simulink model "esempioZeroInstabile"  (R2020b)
settings: Solver=FixedStepAuto  StartTime=0.0  StopTime=30  FixedStep=0.01  RelTol=1e-3

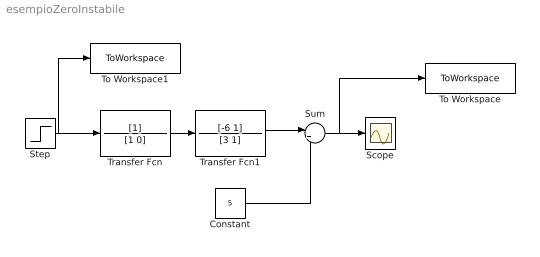
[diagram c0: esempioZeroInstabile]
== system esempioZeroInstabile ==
  Constant : Constant  Value=5
  Scope : Scope
  Step : Step  Time=10  SampleTime=0
  Sum : Sum  Inputs=|++
  To Workspace : ToWorkspace  VariableName=y  SaveFormat=Timeseries  SampleTime=-1
  To Workspace1 : ToWorkspace  VariableName=u  SaveFormat=Timeseries  SampleTime=-1
  Transfer Fcn : TransferFcn  Denominator=[1 0]
  Transfer Fcn1 : TransferFcn  Numerator=[-6 1]  Denominator=[3 1]
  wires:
  Step/1 -> To Workspace1/1, Transfer Fcn/1
  Transfer Fcn/1 -> Transfer Fcn1/1
  Transfer Fcn1/1 -> Sum/1
  Constant/1 -> Sum/2
  Sum/1 -> To Workspace/1, Scope/1
